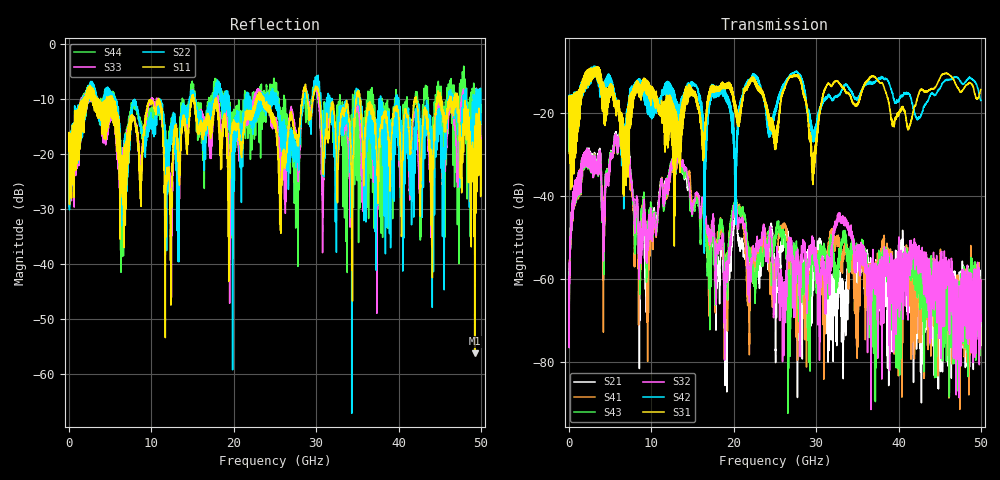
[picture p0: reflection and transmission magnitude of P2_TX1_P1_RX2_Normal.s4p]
!Keysight Technologies,N5225B,MY57041031,A.13.20.10
!Date: Friday, May 31, 2019 11:16:17
!Correction: S11(Full 4 Port(1,2,3,4))
!S12(Full 4 Port(1,2,3,4))
!S13(Full 4 Port(1,2,3,4))
!S14(Full 4 Port(1,2,3,4))
!S21(Full 4 Port(1,2,3,4))
!S22(Full 4 Port(1,2,3,4))
!S23(Full 4 Port(1,2,3,4))
!S24(Full 4 Port(1,2,3,4))
!S31(Full 4 Port(1,2,3,4))
!S32(Full 4 Port(1,2,3,4))
!S33(Full 4 Port(1,2,3,4))
!S34(Full 4 Port(1,2,3,4))
!S41(Full 4 Port(1,2,3,4))
!S42(Full 4 Port(1,2,3,4))
!S43(Full 4 Port(1,2,3,4))
!S44(Full 4 Port(1,2,3,4))
!S4P File: Measurements: <S11,S12,S13,S14>,
!<S21,S22,S23,S24>,
!<S31,S32,S33,S34>,
!<S41,S42,S43,S44>:
# Hz S  dB  R 50.0
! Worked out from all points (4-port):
!   5000 points, 10 MHz to 50 GHz, reference 50 ohm
!   strongest paths, dB at 10 MHz, 12.51 GHz, 25.01 GHz, 37.51 GHz, 50 GHz:
!     S31: -19.4, -17.3, -28.7, -12.1, -14.3
!     S42: -19.4, -16.0, -18.9, -11.8, -16.9
!     S32: -59.7, -31.6, -64.1, -60.1, -68.8
!     S43: -58.3, -31.5, -52.0, -57.6, -64.0
!     S41: -58.6, -32.3, -60.2, -57.9, -60.4
!     S21: -62.2, -32.2, -60.2, -60.6, -64.6
!   lowest |S11| = -56.3 dB at 49.25 GHz (marker M1), VSWR 1.00, Z = 49.9 + j0.113 ohm
!   |S11| at or under -10 dB: 5.36 GHz to 10.81 GHz (5.45 GHz wide, 67.4 % of centre); 17.89 GHz to 22.7 GHz (4.806 GHz wide, 23.7 % of centre); 35.31 GHz to 41.96 GHz (6.644 GHz wide, 17.2 % of centre)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
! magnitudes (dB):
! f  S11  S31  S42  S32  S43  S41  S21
! 10 MHz  -19.5  -19.4  -19.4  -59.7  -58.3  -58.6  -62.2
! 1.77 GHz  -14.0  -14.9  -14.9  -30.1  -30.5  -30.5  -30.1
! 6.39 GHz  -23.7  -25.4  -32.7  -24.5  -24.2  -24.8  -24.5
! 8.52 GHz  -22.8  -13.0  -13.3  -60.1  -49.5  -51.0  -54.3
! 19.03 GHz  -14.0  -13.0  -15.1  -58.4  -57.4  -55.5  -64.0
! 49.25 GHz  -56.3  -15.3  -12.4  -63.0  -62.2  -64.4  -63.9
! 50 GHz  -17.5  -14.3  -16.9  -68.8  -64.0  -60.4  -64.6
